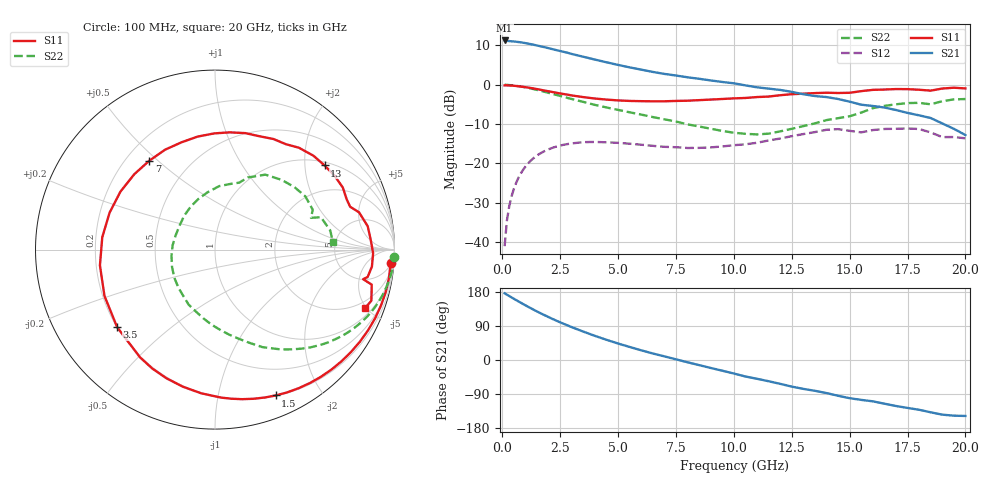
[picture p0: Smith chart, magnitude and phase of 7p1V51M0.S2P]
! Infineon Technologies  Discrete & RF Semiconductors
! bfp620
! VCE =  1.5 V,  IC =  1.0 mA
! Common Emitter S-Parameters:  Sep 2002
# GHz  S  MA  R  50
!  f  S11  S21  S12  S22
! GHz  MAG  ANG  MAG  ANG  MAG  ANG  MAG  ANG
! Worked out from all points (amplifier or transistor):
!   59 points, 100 MHz to 20 GHz, reference 50 ohm
!   highest |S21| = 11.3 dB at 100 MHz (marker M1)
!   |S21| within 3 dB of that: start of sweep to 2.725 GHz
!   unconditionally stable (mu >= 1): 6.36 GHz to 15.78 GHz; 17.78 GHz to end of sweep
!   at 1 GHz: K = 0.10, MSG = 15.7 dB, |S12| = -20.8 dB
!   at 5.5 GHz: K = 0.82, MSG = 9.7 dB, |S12| = -15.0 dB
!   at 20 GHz: K = 1.46, MAG = -3.6 dB, |S12| = -13.6 dB
!   S11 on the Smith chart (normalised r, x): 100 MHz: 6, -24; 1.5 GHz: 0.20, -1.48; 3.5 GHz: 0.20, -0.34; 7 GHz: 0.29, +0.47; 13 GHz: 1.10, +2.52; 20 GHz: 1.47, -4.92
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0.1  0.9816 -4.5  3.665 176.0  0.0088 86.1  1 -2.5
0.2  0.9821 -9.3  3.624 172.4  0.0187 84.6  0.9963 -5.1
0.5  0.9705 -23.3  3.554 161.6  0.0473 76.5  0.9774 -12.4
1  0.9314 -45.9  3.39 144.3  0.0908 61.4  0.9259 -23.8
1.5  0.8804 -67.4  3.162 128.1  0.1256 47.6  0.8586 -33.8
1.9  0.8359 -83.7  2.97 116.1  0.1464 37.9  0.8023 -40.9
2.4  0.7847 -103.1  2.732 102.1  0.1653 27.1  0.7342 -48.7
3  0.7313 -124.8  2.465 86.7  0.1792 15.7  0.6584 -57.4
3.5  0.6958 -141.6  2.273 74.9  0.1859 7.4  0.6048 -64.0
4  0.6676 -157.3  2.092 63.7  0.187 -0.4  0.554 -69.7
5  0.6319 173.8  1.79 43.5  0.182 -11.7  0.4787 -80.8
6  0.618 148.5  1.558 25.6  0.1723 -20.0  0.4168 -93.0
7  0.6158 126.5  1.375 9.6  0.162 -24.5  0.3629 -106.6
8.5  0.6369 98.8  1.191 -13.5  0.1571 -26.8  0.2941 -133.9
10.5  0.6788 68.3  0.982 -43.5  0.1744 -30.1  0.2373 174.0
13  0.7697 37.5  0.758 -76.2  0.2354 -41.6  0.2972 108.0
13.5  0.783 31.7  0.718 -81.3  0.2495 -46.2  0.3225 97.2
15  0.7899 17.6  0.609 -100.8  0.2591 -67.0  0.3968 70.1
16  0.8608 8.7  0.537 -109.0  0.2647 -70.1  0.5031 56.1
17  0.8812 -1.3  0.477 -121.4  0.275 -82.3  0.5634 38.1
18.5  0.8417 -11.3  0.377 -138.0  0.2472 -105.4  0.5634 18.3
20  0.8976 -21.2  0.229 -147.7  0.208 -110.9  0.658 3.9
